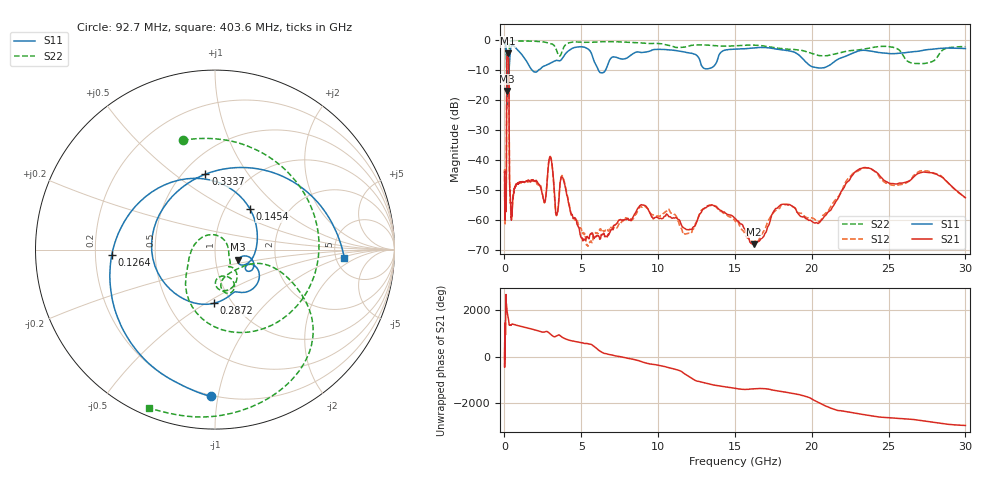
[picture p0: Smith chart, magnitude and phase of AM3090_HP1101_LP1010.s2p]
! Date/Time: Thu, Feb 28, 2019 2:08 PM
! Network Analyzer: Agilent Technologies E8364B Rev: A.07.50.67
! Sweep from 0.010 to 30.000 GHz, 1601 Points, Sweep Type: LOG
! Power Supply: 5.022 V, 0.002 A
# Hz S DB R 50
!freq MagS11 AngS11 MagS21 AngS21 MagS12 AngS12 MagS22 AngS22
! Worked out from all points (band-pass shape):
!   1601 points, 10 MHz to 30 GHz, reference 50 ohm
!   highest |S21| = -4.48 dB at 201.3 MHz (marker M1); lowest = -68.1 dB at 16.21 GHz (marker M2)
!   |S21| within 3 dB of the highest: 152.3 MHz to 275.3 MHz (123 MHz wide, 57.5 % of centre)
!   lowest |S11| = -17.0 dB at 174.1 MHz (marker M3), VSWR 1.33, Z = 64.3 - j7.41 ohm
!   |S11| at or under -10 dB: 144.2 MHz to 293.2 MHz (149 MHz wide, 68.1 % of centre); 1.793 GHz to 2.228 GHz (435.4 MHz wide, 21.7 % of centre); 6.11 GHz to 6.584 GHz (473.8 MHz wide, 7.47 % of centre)
!   |S22| runs from -22.7 to -0.2 dB; largest |S21 - S12| = 0.012
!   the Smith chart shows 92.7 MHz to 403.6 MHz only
!   S11 on the Smith chart (normalised r, x): 92.7 MHz: 0.19, -0.95; 126.4 MHz: 0.27, -0.03; 145.4 MHz: 1.30, +0.65; 287.2 MHz: 0.83, -0.54; 333.7 MHz: 0.64, +0.65; 403.6 MHz: 5.94, -1.20
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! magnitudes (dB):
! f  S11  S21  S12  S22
! 10 MHz  -0.3  -44.2  -43.9  -0.6
! 38.04 MHz  -0.4  -55.9  -55.7  -1.4
! 92.7 MHz  -1.7  -53.1  -53.4  -4.0
! 126.4 MHz  -4.8  -40.7  -40.5  -5.2
! 144.7 MHz  -10.2  -11.8  -11.7  -19.4
! 145.4 MHz  -10.5  -11.2  -11.1  -20.1
! 174.1 MHz  -17.0  -4.9  -4.8  -16.8
! 201.3 MHz  -12.6  -4.5  -4.5  -12.7
! 287.2 MHz  -10.5  -11.1  -11.1  -10.8
! 333.7 MHz  -7.5  -47.4  -47.5  -1.0
! 403.6 MHz  -2.8  -54.8  -56.1  -0.4
! 550.5 MHz  -2.0  -52.9  -52.4  -0.3
! 2.084 GHz  -10.7  -47.0  -47.7  -0.5
! 2.61 GHz  -8.7  -54.2  -54.2  -0.7
! 2.987 GHz  -7.7  -39.0  -38.9  -1.2
! 3.385 GHz  -6.8  -58.5  -58.6  -3.4
! 3.798 GHz  -5.9  -46.0  -45.7  -3.2
! 5.473 GHz  -3.1  -66.0  -67.9  -0.8
! 7.926 GHz  -6.1  -59.9  -59.5  -0.8
! 16.21 GHz  -2.6  -68.1  -67.4  -1.7
! 23.36 GHz  -3.4  -42.6  -42.8  -3.1
! 30 GHz  -2.9  -52.6  -52.7  -2.2
